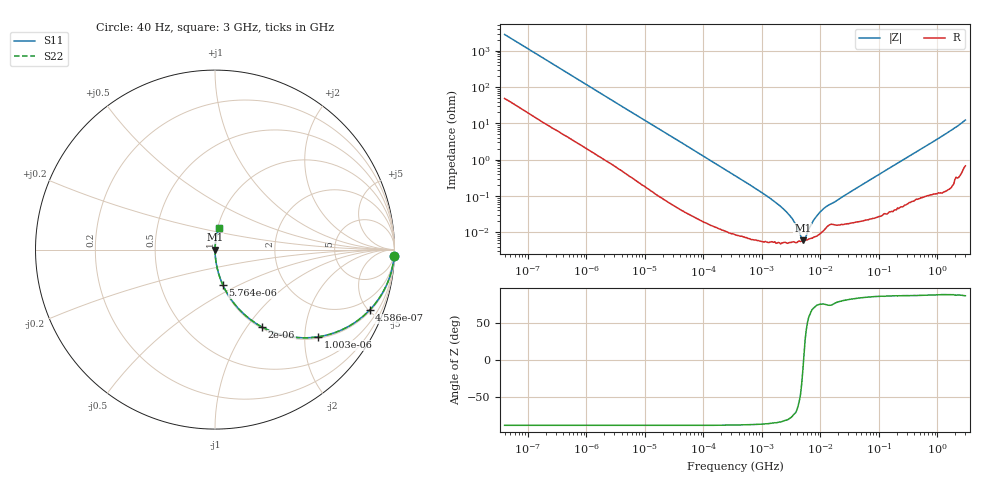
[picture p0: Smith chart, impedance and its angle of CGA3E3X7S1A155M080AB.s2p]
! S-Parameter Data Generated by TDK Corporation
! Copyright(C) 2019 TDK Corporation.
! All Rights Reserved.
! TDK P/N: CGA3E3X7S1A155M080AB (Multilayer Ceramic Chip Capacitor)
! Property: C=1.5uF
! Size(LxWxT): 1.6x0.8x0.8mm
! Model Type: s2p (Touchstone File Format Version 1.0)
! Frequency: DC=Yes Start=4E-05MHz Stop=3000MHz 396points Log-sweep
! Model Generated on July 26, 2019
! Port Assignments:
!  1 ---| |--- 2
! Applicable Conditions:
!  Temperature = 25 degC
!  DC Bias Voltage = 0 V
!  Small Signal Operation
! Terms and conditions regarding TDK Simulation Models
! (1)This simulation model is being provided solely for informational purposes. Please refer to the specifications of the products in terms of detailed characteristics of such products.
! (2)In no event shall TDK Corporation of any of its subsidiaries be liable for any loss or damage arising, directly or indirectly,
!  From any information contained in this simulation model, including, but not limited to loss or damages arising from any inaccuracies, omissions or errors in connection with such information.
! (3)Any and all copyrights on this simulation model are owned by TDK Corporation.
!  Duplication or redistribution of this simulation model without prior written permission from TDK Corporation is prohibited.
! (4)This simulation model is subject to any modification or change without any prior notice.
! (5)Neither TDK Corporation nor any of its subsidiaries shall make any warranty, express or implied,
!  Including but not limited to the correctness, implied warranties of merchantability and fitness for a particular purpose with respect to this simulation models.
! (6)The use of this simulation model shall be deemed to have consented to the terms and conditions hereof.
# Hz S MA R 50
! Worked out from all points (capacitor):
!   395 points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, 40 Hz to 3 GHz, reference 50 ohm
!   read as one part in series: C = 1.4 uF near 41.88 Hz
!   lowest |Z| = 6.01 mohm at 4.999 MHz (marker M1)
!   series resonance near 5.156 MHz, so ESL is about 680 pH
!   S11 on the Smith chart (normalised r, x): 40 Hz: 2, -56; 458.6 Hz: 1.09, -5.07; 1.003 kHz: 1.04, -2.33; 2 kHz: 1.02, -1.18; 5.764 kHz: 1.01, -0.42; 3 GHz: 1.01, +0.25
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40  0.9988 -2.0  0.03536 87.0  0.03536 87.0  0.9988 -2.0
151.9485  0.9892 -7.5  0.1307 81.5  0.1307 81.5  0.9892 -7.5
458.5594  0.9247 -21.4  0.365 67.6  0.365 67.6  0.9247 -21.4
834.128  0.8071 -35.2  0.5766 53.8  0.5766 53.8  0.8071 -35.2
1002.727  0.7528 -40.2  0.6454 48.8  0.6454 48.8  0.7528 -40.2
1999.837  0.504 -58.8  0.8551 30.3  0.8551 30.3  0.504 -58.8
3317.849  0.3352 -69.5  0.9366 19.6  0.9366 19.6  0.3352 -69.5
5763.764  0.2031 -77.4  0.9759 11.7  0.9759 11.7  0.2031 -77.4
17394.24  0.07032 -85.2  0.9966 4.0  0.9966 4.0  0.07032 -85.2
346410.2  0.003658 -88.4  0.9999 0.2  0.9999 0.2  0.003658 -88.4
1146211  0.001066 -86.9  0.9999 0.1  0.9999 0.1  0.001066 -86.9
2084979  0.0005182 -84.7  1 0.0  1 0.0  0.0005182 -84.7
3303516  0.0002369 -76.8  0.9999 0.0  0.9999 0.0  0.0002369 -76.8
4354128  0.000103 -55.8  0.9999 0.0  0.9999 0.0  0.000103 -55.8
4998775  6.007e-05 -14.4  0.9999 0.0  0.9999 0.0  6.007e-05 -14.4
6009156  9.865e-05 51.0  0.9999 -0.0  0.9999 -0.0  9.865e-05 51.0
7223760  0.0001845 68.1  0.9999 -0.0  0.9999 -0.0  0.0001845 68.1
9521122  0.0003385 75.1  0.9999 -0.0  0.9999 -0.0  0.0003385 75.1
1.254911e7  0.0005118 74.9  0.9999 -0.0  0.9999 -0.0  0.0005118 74.9
1.506385e8  0.005863 86.1  0.9996 -0.3  0.9996 -0.3  0.005863 86.1
1.040901e9  0.03859 86.0  0.998 -2.2  0.998 -2.2  0.03859 86.0
3e9  0.1224 79.9  0.9858 -7.0  0.9858 -7.0  0.1224 79.9
